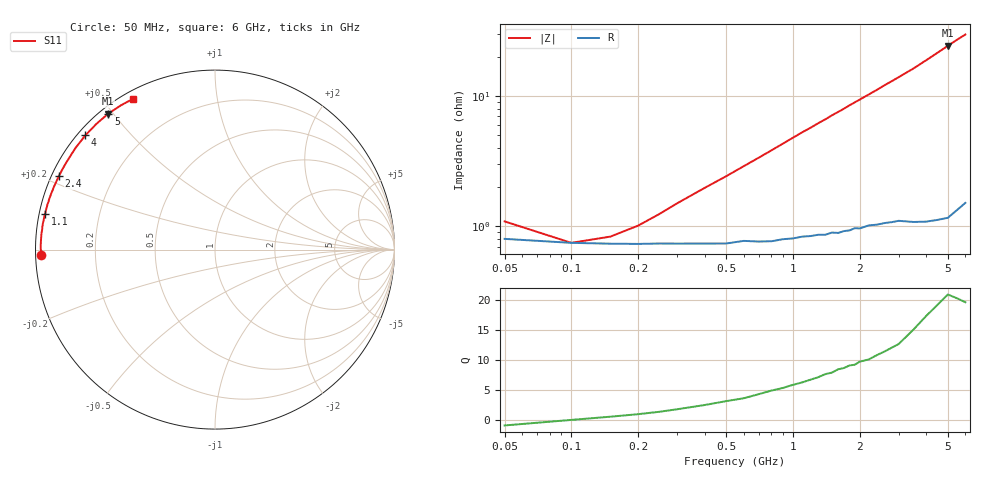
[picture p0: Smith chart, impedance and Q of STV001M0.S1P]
! SIEMENS Discrete & RF Semiconductors
! BA892
! Si PIN Diode in SCD-80
! IF = 1 mA
! S-Parameters:  September  1997
# GHz  S  MA  R  50
!  f  S11
! GHz  MAG  ANG
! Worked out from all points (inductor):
!   34 points, 50 MHz to 6 GHz, reference 50 ohm
!   read as one part to ground: L = 745 pH near 500 MHz
!   highest Q = 20.3 at 5 GHz (marker M1), where L = 774 pH
!   S11 on the Smith chart (normalised r, x): 50 MHz: 0.02, -0.01; 1.1 GHz: 0.02, +0.10; 2.4 GHz: 0.02, +0.22; 4 GHz: 0.02, +0.38; 5 GHz: 0.02, +0.49; 6 GHz: 0.03, +0.59
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0.05  0.9684 -178.3
0.1  0.9706 -180.0
0.15  0.971 179.1
0.3  0.9709 177.0
0.4  0.9709 175.8
0.5  0.9709 174.7
0.6  0.9696 173.6
0.8  0.9699 171.4
1.1  0.9675 168.1
1.2  0.9673 167.1
1.3  0.9666 166.0
1.4  0.9667 165.0
1.5  0.9655 163.9
1.6  0.9658 162.9
1.7  0.9647 161.9
1.8  0.9644 160.8
1.9  0.9631 159.8
2  0.9634 158.8
2.4  0.9615 154.8
2.6  0.9607 152.7
2.8  0.9604 150.8
3  0.9599 148.8
3.5  0.9617 143.9
4  0.9626 138.6
4.5  0.9629 133.3
5  0.963 128.1
5.5  0.9595 123.1
6  0.9562 118.5
